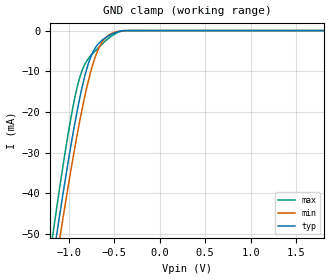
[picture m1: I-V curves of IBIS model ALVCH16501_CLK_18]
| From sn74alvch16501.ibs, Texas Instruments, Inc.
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[Model]   ALVCH16501_CLK_18
Model_type  Input
Vinl=0.5775
Vinh=1.2675
| variable   typ   min   max
C_comp   1.11pF   0.85pF   1.23pF
[Temperature Range]   40   100   -40
| Ambient temperature   25   85   -40
[Voltage range]   1.8   1.65   1.95
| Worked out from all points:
|   GND clamp passes 1 mA (typ) near -0.53 V on its own axis
[GND Clamp]
| ALVCH16501_CLK_18
|   Voltage   I(typ)   I(min)   I(max)
-1.8V     -157.3mA   -159.8mA   -155.7mA
-1.17V    -56.16mA   -61.76mA   -49.84mA
-1.12V    -48.72mA   -54.5mA    -42.11mA
-1.09V    -44.35mA   -50.22mA   -37.59mA
-960mV    -26.48mA   -32.51mA   -19.81mA
-865mV    -15.36mA   -20.9mA    -10.69mA
-785mV    -8.33mA    -12.59mA   -6.976mA
-705mV    -4.213mA   -6.363mA   -4.971mA
-635mV    -2.431mA   -2.986mA   -3.388mA
-555mV    -1.254mA   -1.07mA    -1.791mA
-375mV    -1.864uA   -31.43uA   -304.7nA
1.8V      909pA      48.34nA    11.01pA
